(* Logix 5000 AddOnInstructionDefinition export SPEL_PointSet; software revision 30.01 *)

ADD_ON_INSTRUCTION SPEL_ExecCmd   (* revision 1.2 *)
// Executes a command in the robot controller.  Normally this is called by higher level AOIs.
VAR_INPUT
   Start : BOOL; {required}
   MaxTime : DINT := 3000; {required}
END_VAR
VAR_OUTPUT
   InCycle : BOOL; {access Read Only, visible}
   Done : BOOL; {access Read Only, visible}
   Error : BOOL; {access Read Only, visible}
END_VAR
VAR_IN_OUT
   ExtInputs : AB:ETHERNET_MODULE_INT_128Bytes:I:0; {required}
        .DATA[0].0   // ExtCmdGet
        .DATA[0].1   // ExtRespSet
        .DATA[0].2   // ExtCmdResult
        .DATA[0].3   // ExtError
   ExtOutputs : AB:ETHERNET_MODULE_INT_128Bytes:O:0; {required}
        .DATA[0].0   // ExtCmdSet
        .DATA[0].1   // ExtRespGet
        .DATA[0].2   // ExtCmdReset
END_VAR
VAR_INPUT
   Cmd : INT; {required}
   CmdParam1 : INT; {required}
   CmdParam2 : INT; {required}
   CmdParam3 : INT; {required}
   CmdParam4 : INT; {required}
   CmdParam5 : INT; {required}
   CmdParam6 : INT; {required}
   CmdParam7 : INT; {required}
END_VAR
VAR_OUTPUT
   CmdEcho : INT; {access Read Only, visible}
   Resp1 : INT; {access Read Only, visible}
   Resp2 : INT; {access Read Only, visible}
   Resp3 : INT; {access Read Only, visible}
   Resp4 : INT; {access Read Only, visible}
   Resp5 : INT; {access Read Only, visible}
   Resp6 : INT; {access Read Only, visible}
   Resp7 : INT; {access Read Only, visible}
   ErrCode1 : INT; {access Read Only, visible}
   ErrCode2 : INT; {access Read Only, visible}
END_VAR
VAR
   ExtReset : BOOL; {access None}
   ExtError : BOOL; {access None}
   ExtCmdSet : BOOL; {access None}   // Cmd Ready
   ExtCmdGet : BOOL; {access None}   // Cmd Received
   CmdXferDone : BOOL; {access None}
   ExtRespSet : BOOL; {access None}   // Resp Ready
   RespXferDone : BOOL; {access None}
   ExtCmdResult : BOOL; {access None}   // Normal or Error?
   TmrCmdDataRdy : TIMER := (PRE := 5); {access None}
   OneShotDoneOff : BOOL; {access None}
   OneShotStart : BOOL; {access None}
   StartInit : BOOL; {access None}
   OneShotStartError : BOOL; {access None}
   TmrCycle : TIMER := (PRE := 5000); {access None}
   OneshotTmrPreset : BOOL; {access None}
   TmrCmdSet : TIMER := (PRE := 20); {access None}
   OnShotCmdDataXfer : BOOL; {access None}
   OneShotRespDataXfer : BOOL; {access None}
   OneShotDataRdy : BOOL; {access None}
   OtherCmdInCycle : BOOL; {access None}
   s : BOOL; {access None}
   OneShotUnsetCmdIncycle : BOOL; {access None}
   OneShotSetCmdIncycle : BOOL; {access None}
   OneShotSetOtherCmdInCycleError : BOOL; {access None}
   OneShotSetBit : BOOL; {access None}
   MaxTimeError : BOOL; {access None}
END_VAR

ROUTINE Logic   (* ladder *)
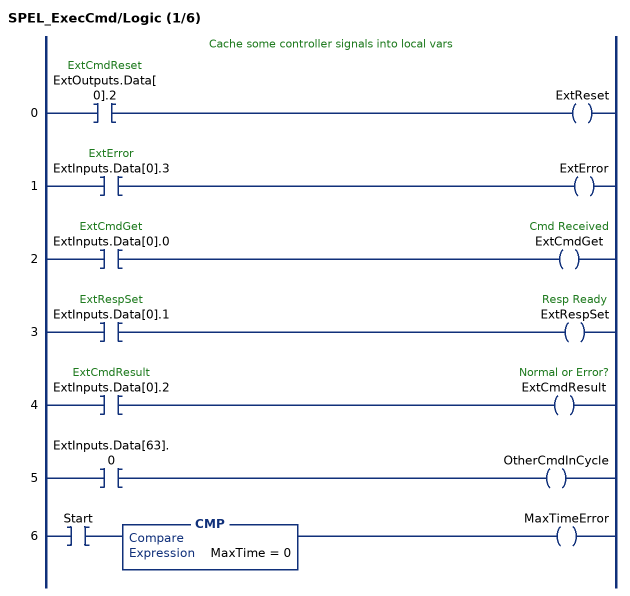
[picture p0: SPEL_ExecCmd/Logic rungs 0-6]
   // Cache some controller signals into local vars
   0: XIC(ExtOutputs.Data[0].2)OTE(ExtReset);
   1: XIC(ExtInputs.Data[0].3)OTE(ExtError);
   2: XIC(ExtInputs.Data[0].0)OTE(ExtCmdGet);
   3: XIC(ExtInputs.Data[0].1)OTE(ExtRespSet);
   4: XIC(ExtInputs.Data[0].2)OTE(ExtCmdResult);
   5: XIC(ExtInputs.Data[63].0)OTE(OtherCmdInCycle);
   6: XIC(Start)CMP(MaxTime = 0)OTE(MaxTimeError);
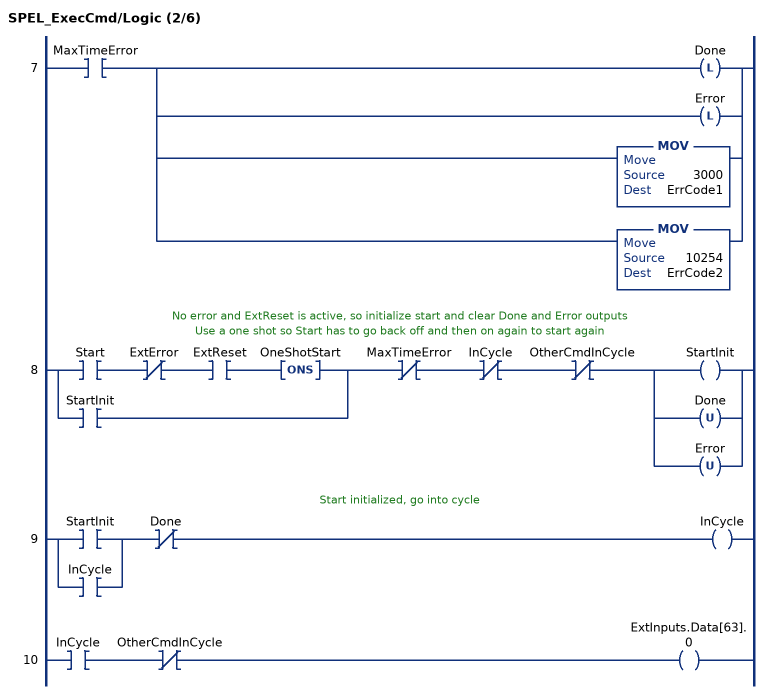
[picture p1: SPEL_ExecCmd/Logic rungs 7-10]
   7: XIC(MaxTimeError)[OTL(Done) ,OTL(Error) ,MOV(3000,ErrCode1) ,MOV(10254,ErrCode2) ];
   // No error and ExtReset is active, so initialize start and clear Done and Error outputs
   // Use a one shot so Start has to go back off and then on again to start again
   8: [XIC(Start) XIO(ExtError) XIC(ExtReset) ONS(OneShotStart) ,XIC(StartInit) ]XIO(MaxTimeError)XIO(InCycle)XIO(OtherCmdInCycle)[OTE(StartInit) ,OTU(Done) ,OTU(Error) ];
   // Start initialized, go into cycle
   9: [XIC(StartInit) ,XIC(InCycle) ]XIO(Done)OTE(InCycle);
   10: XIC(InCycle)XIO(OtherCmdInCycle)OTE(ExtInputs.Data[63].0);
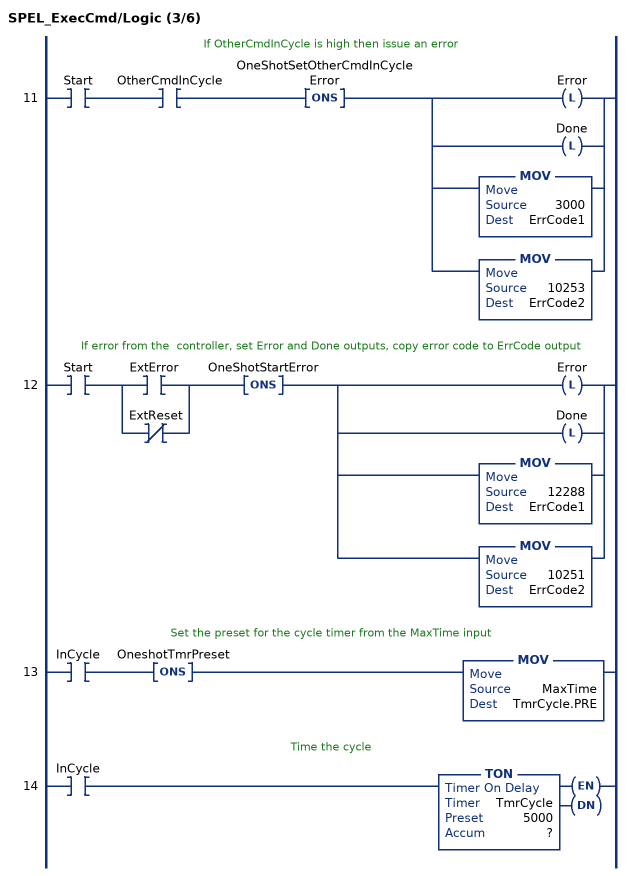
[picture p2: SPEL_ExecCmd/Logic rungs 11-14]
   // If OtherCmdInCycle is high then issue an error
   11: XIC(Start)XIC(OtherCmdInCycle)ONS(OneShotSetOtherCmdInCycleError)[OTL(Error) ,OTL(Done) ,MOV(3000,ErrCode1) ,MOV(10253,ErrCode2) ];
   // If error from the  controller, set Error and Done outputs, copy error code to ErrCode output
   12: XIC(Start)[XIC(ExtError) ,XIO(ExtReset) ]ONS(OneShotStartError)[OTL(Error) ,OTL(Done) ,MOV(12288,ErrCode1) ,MOV(10251,ErrCode2) ];
   // Set the preset for the cycle timer from the MaxTime input
   13: XIC(InCycle)ONS(OneshotTmrPreset)MOV(MaxTime,TmrCycle.PRE);
   // Time the cycle
   14: XIC(InCycle)TON(TmrCycle,?,?);
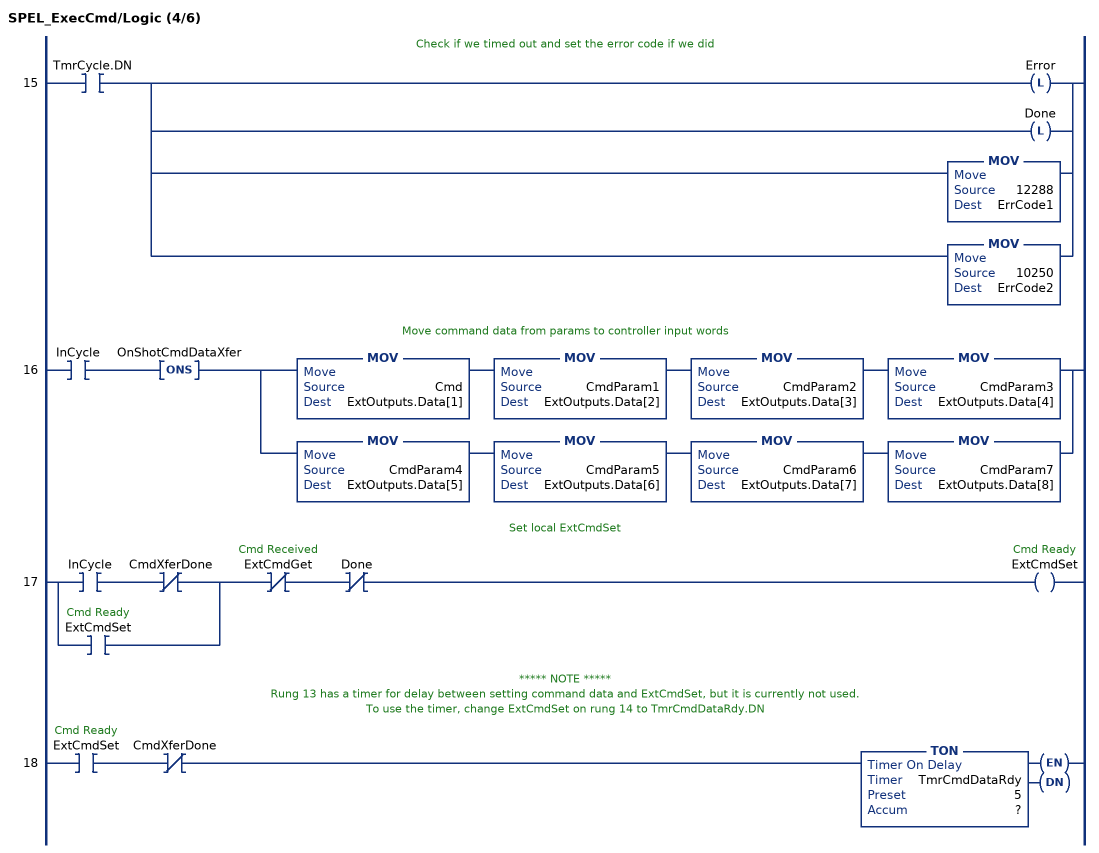
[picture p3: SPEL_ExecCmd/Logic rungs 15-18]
   // Check if we timed out and set the error code if we did
   15: XIC(TmrCycle.DN)[OTL(Error) ,OTL(Done) ,MOV(12288,ErrCode1) ,MOV(10250,ErrCode2) ];
   // Move command data from params to controller input words
   16: XIC(InCycle)ONS(OnShotCmdDataXfer)[MOV(Cmd,ExtOutputs.Data[1]) MOV(CmdParam1,ExtOutputs.Data[2]) MOV(CmdParam2,ExtOutputs.Data[3]) MOV(CmdParam3,ExtOutputs.Data[4]) ,MOV(CmdParam4,ExtOutputs.Data[5]) MOV(CmdParam5,ExtOutputs.Data[6]) MOV(CmdParam6,ExtOutputs.Data[7]) MOV(CmdParam7,ExtOutputs.Data[8]) ];
   // Set local ExtCmdSet
   17: [XIC(InCycle) XIO(CmdXferDone) ,XIC(ExtCmdSet) ]XIO(ExtCmdGet)XIO(Done)OTE(ExtCmdSet);
   // ***** NOTE *****
   // Rung 13 has a timer for delay between setting command data and ExtCmdSet, but it is currently not used.
   // To use the timer, change ExtCmdSet on rung 14 to TmrCmdDataRdy.DN
   18: XIC(ExtCmdSet)XIO(CmdXferDone)TON(TmrCmdDataRdy,?,?);
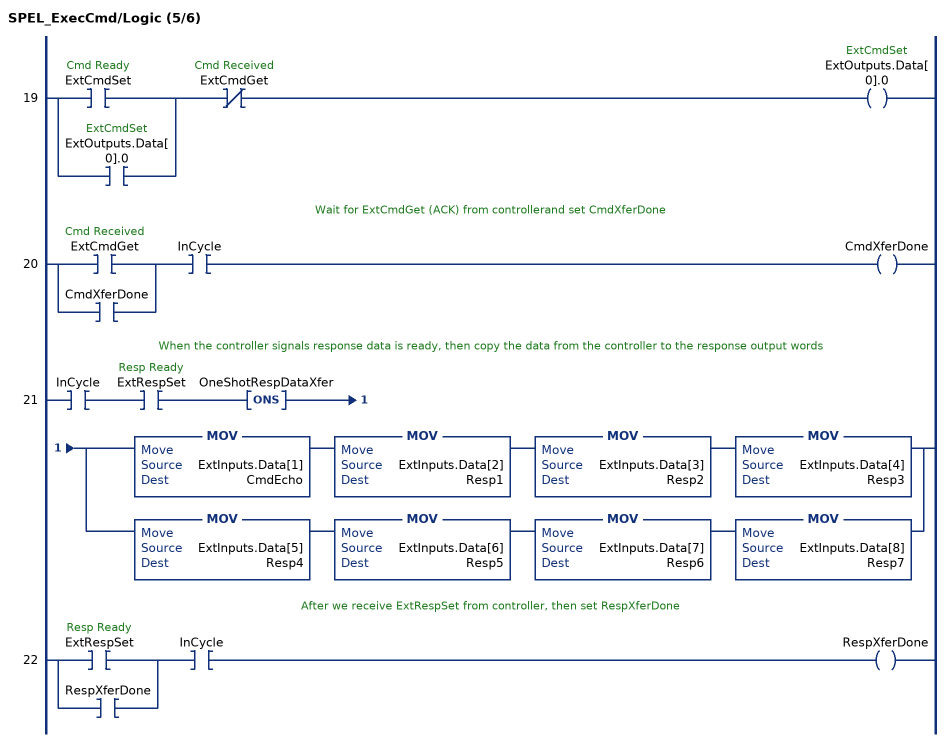
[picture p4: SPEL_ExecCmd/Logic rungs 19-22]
   19: [XIC(ExtCmdSet) ,XIC(ExtOutputs.Data[0].0) ]XIO(ExtCmdGet)OTE(ExtOutputs.Data[0].0);
   // Wait for ExtCmdGet (ACK) from controllerand set CmdXferDone
   20: [XIC(ExtCmdGet) ,XIC(CmdXferDone) ]XIC(InCycle)OTE(CmdXferDone);
   // When the controller signals response data is ready, then copy the data from the controller to the response output words
   21: XIC(InCycle)XIC(ExtRespSet)ONS(OneShotRespDataXfer)[MOV(ExtInputs.Data[1],CmdEcho) MOV(ExtInputs.Data[2],Resp1) MOV(ExtInputs.Data[3],Resp2) MOV(ExtInputs.Data[4],Resp3) ,MOV(ExtInputs.Data[5],Resp4) MOV(ExtInputs.Data[6],Resp5) MOV(ExtInputs.Data[7],Resp6) MOV(ExtInputs.Data[8],Resp7) ];
   // After we receive ExtRespSet from controller, then set RespXferDone
   22: [XIC(ExtRespSet) ,XIC(RespXferDone) ]XIC(InCycle)OTE(RespXferDone);
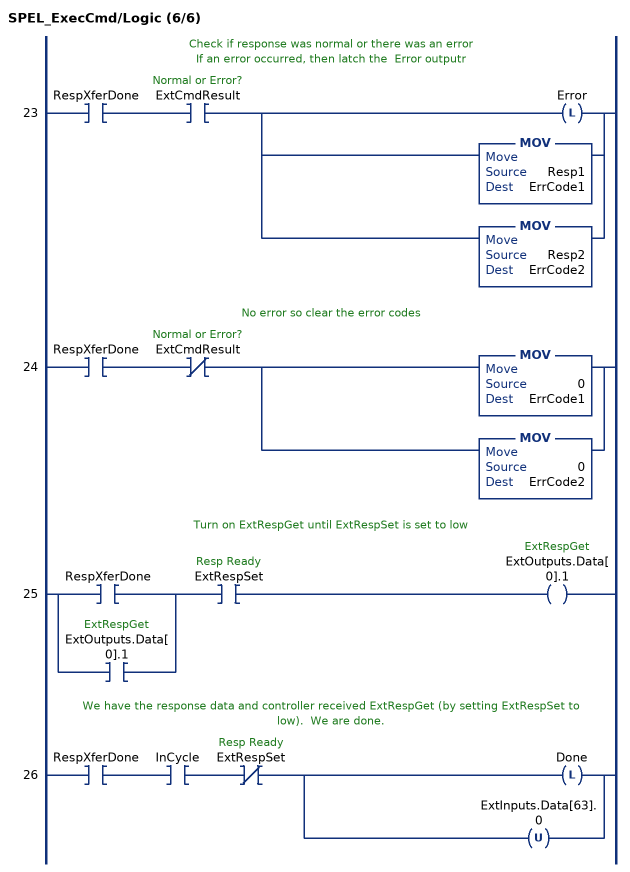
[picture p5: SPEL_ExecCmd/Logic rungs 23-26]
   // Check if response was normal or there was an error
   // If an error occurred, then latch the  Error outputr
   23: XIC(RespXferDone)XIC(ExtCmdResult)[OTL(Error) ,MOV(Resp1,ErrCode1) ,MOV(Resp2,ErrCode2) ];
   // No error so clear the error codes
   24: XIC(RespXferDone)XIO(ExtCmdResult)[MOV(0,ErrCode1) ,MOV(0,ErrCode2) ];
   // Turn on ExtRespGet until ExtRespSet is set to low
   25: [XIC(RespXferDone) ,XIC(ExtOutputs.Data[0].1) ]XIC(ExtRespSet)OTE(ExtOutputs.Data[0].1);
   // We have the response data and controller received ExtRespGet (by setting ExtRespSet to low).  We are done.
   26: XIC(RespXferDone)XIC(InCycle)XIO(ExtRespSet)[OTL(Done) ,OTU(ExtInputs.Data[63].0) ];
END_ROUTINE
END_ADD_ON_INSTRUCTION

ADD_ON_INSTRUCTION SPEL_PointSet   (* revision 1.2, vendor SEIKO EPSON CORP. *)
// Sets the specified coordinate value to the coordinate of specified axes.
VAR_OUTPUT
   InCycle : BOOL; {access Read Only, visible}
   Done : BOOL; {access Read Only, visible}
   Error : BOOL; {access Read Only, visible}
END_VAR
VAR_INPUT
   Start : BOOL; {access None, required}
   Point : INT; {access None, required}
   X : REAL; {access None, required}
   Y : REAL; {access None, required}
   Z : REAL; {access None, required}
   U : REAL; {access None, required}
   V : REAL; {access None, visible}
   W : REAL; {access None, visible}
END_VAR
VAR_IN_OUT
   ExtInputs : AB:ETHERNET_MODULE_INT_128Bytes:I:0; {required}
   ExtOutputs : AB:ETHERNET_MODULE_INT_128Bytes:O:0; {required}
END_VAR
VAR_OUTPUT
   ErrCode1 : INT; {access Read Only, visible}
   ErrCode2 : INT; {access Read Only, visible}
END_VAR
VAR
   OneShotInit : BOOL[32]; {access None}
   StartInit : BOOL[32]; {access None}
   ExecSetXY : SPEL_ExecCmd := (MaxTime := 3000); {access None}
   CoordinateX1000 : DINT; {access None}
   CoordinateX_INTS : INT[2]; {access None}
   CoordinateY_INTS : INT[2]; {access None}
   CoordinateY1000 : DINT; {access None}
   CoordinateZ1000 : DINT; {access None}
   CoordinateZ_INTS : INT[2]; {access None}
   CoordinateU1000 : DINT; {access None}
   CoordinateU_INTS : INT[2]; {access None}
   ExecSetZU : SPEL_ExecCmd := (MaxTime := 3000); {access None}
   CoordinateV1000 : DINT; {access None}
   CoordinateV_INTS : INT[2]; {access None}
   CoordinateW1000 : DINT; {access None}
   CoordinateW_INTS : INT[2]; {access None}
   ExecSetVW : SPEL_ExecCmd := (MaxTime := 3000); {access None}
END_VAR

ROUTINE Logic   (* ladder *)
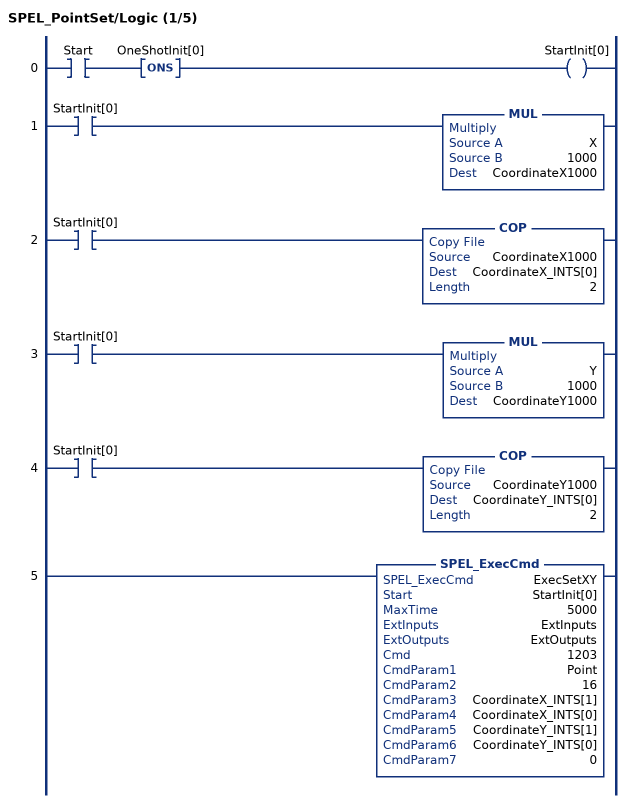
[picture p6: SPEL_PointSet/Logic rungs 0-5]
   0: XIC(Start)ONS(OneShotInit[0])OTE(StartInit[0]);
   1: XIC(StartInit[0])MUL(X,1000,CoordinateX1000);
   2: XIC(StartInit[0])COP(CoordinateX1000,CoordinateX_INTS[0],2);
   3: XIC(StartInit[0])MUL(Y,1000,CoordinateY1000);
   4: XIC(StartInit[0])COP(CoordinateY1000,CoordinateY_INTS[0],2);
   5: SPEL_ExecCmd(ExecSetXY,StartInit[0],5000,ExtInputs,ExtOutputs,1203,Point,16,CoordinateX_INTS[1],CoordinateX_INTS[0],CoordinateY_INTS[1],CoordinateY_INTS[0],0);
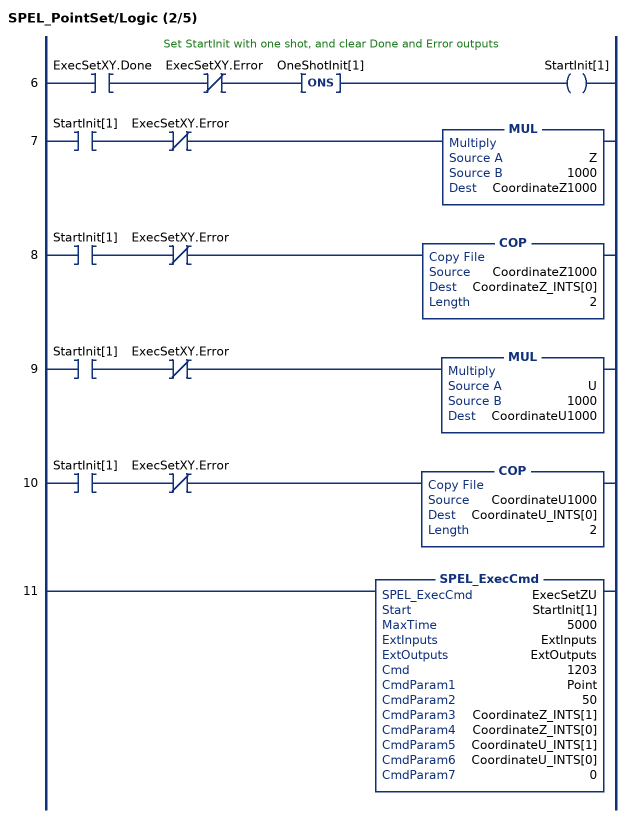
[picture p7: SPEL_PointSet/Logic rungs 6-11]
   // Set StartInit with one shot, and clear Done and Error outputs
   6: XIC(ExecSetXY.Done)XIO(ExecSetXY.Error)ONS(OneShotInit[1])OTE(StartInit[1]);
   7: XIC(StartInit[1])XIO(ExecSetXY.Error)MUL(Z,1000,CoordinateZ1000);
   8: XIC(StartInit[1])XIO(ExecSetXY.Error)COP(CoordinateZ1000,CoordinateZ_INTS[0],2);
   9: XIC(StartInit[1])XIO(ExecSetXY.Error)MUL(U,1000,CoordinateU1000);
   10: XIC(StartInit[1])XIO(ExecSetXY.Error)COP(CoordinateU1000,CoordinateU_INTS[0],2);
   11: SPEL_ExecCmd(ExecSetZU,StartInit[1],5000,ExtInputs,ExtOutputs,1203,Point,50,CoordinateZ_INTS[1],CoordinateZ_INTS[0],CoordinateU_INTS[1],CoordinateU_INTS[0],0);
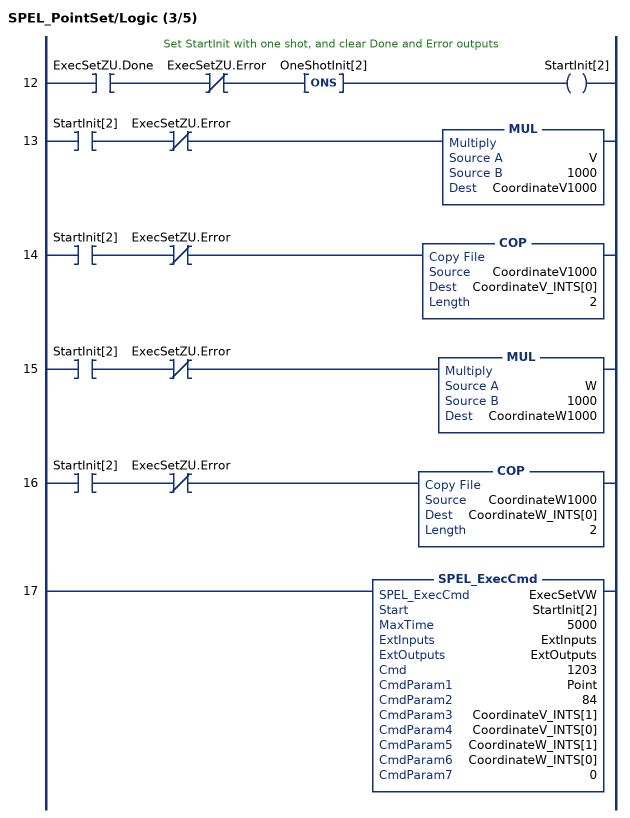
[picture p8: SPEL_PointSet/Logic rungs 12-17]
   // Set StartInit with one shot, and clear Done and Error outputs
   12: XIC(ExecSetZU.Done)XIO(ExecSetZU.Error)ONS(OneShotInit[2])OTE(StartInit[2]);
   13: XIC(StartInit[2])XIO(ExecSetZU.Error)MUL(V,1000,CoordinateV1000);
   14: XIC(StartInit[2])XIO(ExecSetZU.Error)COP(CoordinateV1000,CoordinateV_INTS[0],2);
   15: XIC(StartInit[2])XIO(ExecSetZU.Error)MUL(W,1000,CoordinateW1000);
   16: XIC(StartInit[2])XIO(ExecSetZU.Error)COP(CoordinateW1000,CoordinateW_INTS[0],2);
   17: SPEL_ExecCmd(ExecSetVW,StartInit[2],5000,ExtInputs,ExtOutputs,1203,Point,84,CoordinateV_INTS[1],CoordinateV_INTS[0],CoordinateW_INTS[1],CoordinateW_INTS[0],0);
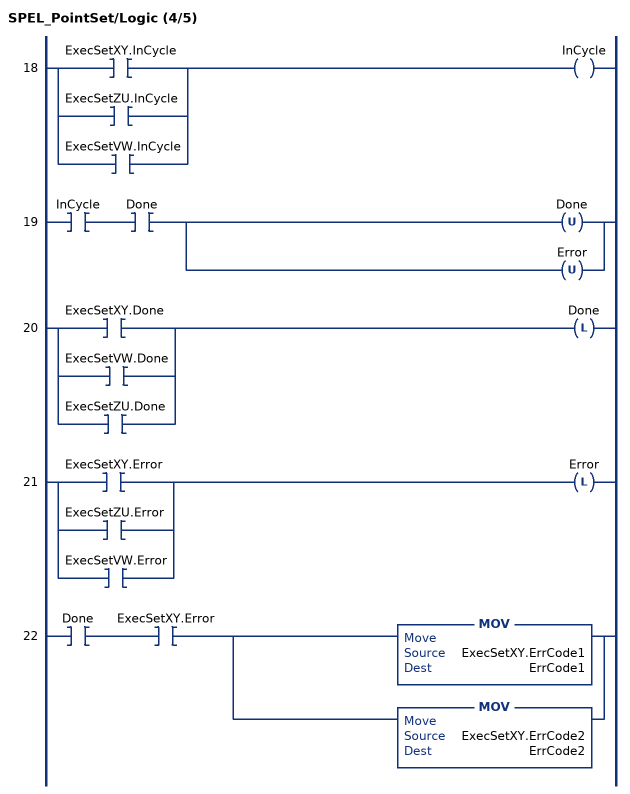
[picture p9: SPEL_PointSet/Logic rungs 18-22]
   18: [XIC(ExecSetXY.InCycle) ,XIC(ExecSetZU.InCycle) ,XIC(ExecSetVW.InCycle) ]OTE(InCycle);
   19: XIC(InCycle)XIC(Done)[OTU(Done) ,OTU(Error) ];
   20: [XIC(ExecSetXY.Done) ,XIC(ExecSetVW.Done) ,XIC(ExecSetZU.Done) ]OTL(Done);
   21: [XIC(ExecSetXY.Error) ,XIC(ExecSetZU.Error) ,XIC(ExecSetVW.Error) ]OTL(Error);
   22: XIC(Done)XIC(ExecSetXY.Error)[MOV(ExecSetXY.ErrCode1,ErrCode1) ,MOV(ExecSetXY.ErrCode2,ErrCode2) ];
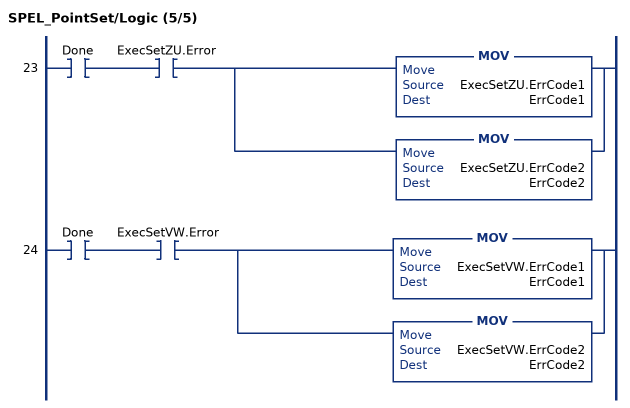
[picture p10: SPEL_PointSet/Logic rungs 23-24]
   23: XIC(Done)XIC(ExecSetZU.Error)[MOV(ExecSetZU.ErrCode1,ErrCode1) ,MOV(ExecSetZU.ErrCode2,ErrCode2) ];
   24: XIC(Done)XIC(ExecSetVW.Error)[MOV(ExecSetVW.ErrCode1,ErrCode1) ,MOV(ExecSetVW.ErrCode2,ErrCode2) ];
END_ROUTINE
END_ADD_ON_INSTRUCTION
